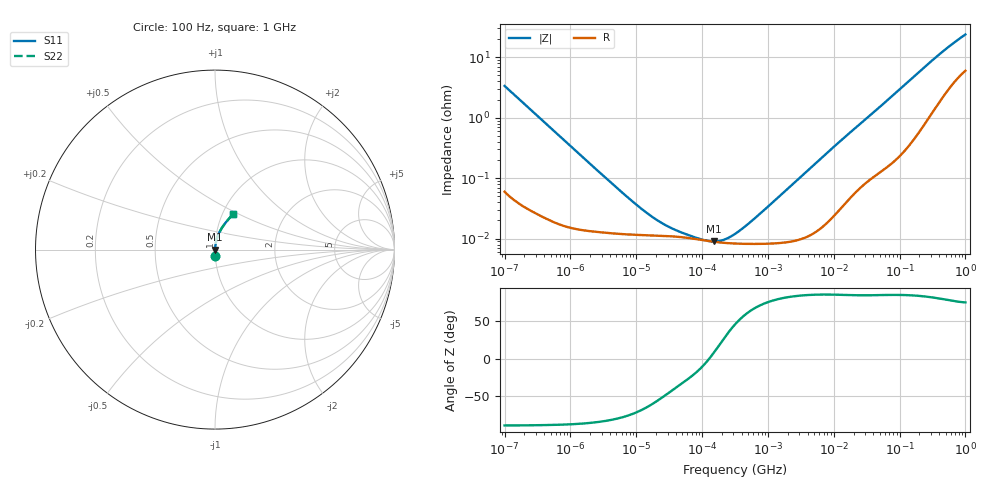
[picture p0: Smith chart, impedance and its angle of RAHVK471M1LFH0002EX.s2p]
! RAHVK471M1LFH0002EX  S-PARAMETER MODEL  (AEC-Q200 qualified)
! Model Generated by ELNA Corporation (http://www.ty-top.com)
! Version 1.0
! ELNA Control No. 201210
! Copyright (c) 2020 ELNA CO.,LTD. All Rights Reserved.
! Products Name : CONDUCTIVE POLYMER HYBRID ALUMINUM ELECTROLYTIC CAPACITORS
! Characteristics :
!  Capacitance  :  470uF  ,  Rated voltage  :  10V
!  Operating Temp. Range  :  -55 to +125 degC  ,  Endurance  :  4000hr at 125 degC
!  Dimension D  :  10mm  ,  Dimension L  :  10mm
! Frequency Range : 100Hz - 1GHz
! External Node Assignments :
!  1  o---| |---o  2
# MHz S RI R 50
!Freq[MHz].  S11 Real  S11 Imag  S21 Real  S21 Imag  S12 Real  S12 Imag  S22 Real  S22 Imag
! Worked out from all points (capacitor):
!   401 points, 100 Hz to 1 GHz, reference 50 ohm
!   read as one part in series: C = 473 uF near 108 Hz
!   lowest |Z| = 8.98 mohm at 153.1 kHz (marker M1)
!   series resonance near 127.7 kHz, so ESL is about 3.3 nH
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0.0001  0.00172 -0.0335  0.9983 0.0335  0.9983 0.0335  0.00172 -0.0335
0.000113  0.00141 -0.0297  0.9986 0.0297  0.9986 0.0297  0.00141 -0.0297
0.000309  0.000376 -0.0109  0.9996 0.0109  0.9996 0.0109  0.000376 -0.0109
0.001488  0.000144 -0.0023  0.9999 0.0023  0.9999 0.0023  0.000144 -0.0023
0.00876  0.000117 -0.000396  0.9999 0.000396  0.9999 0.000396  0.000117 -0.000396
0.014791  0.000114 -0.000235  0.9999 0.000235  0.9999 0.000235  0.000114 -0.000235
0.022131  0.000112 -0.000158  0.9999 0.000158  0.9999 0.000158  0.000112 -0.000158
0.038905  0.000108 -8.88e-05  0.9999 8.88e-05  0.9999 8.88e-05  0.000108 -8.88e-05
0.080353  9.85e-05 -3.3e-05  0.9999 3.3e-05  0.9999 3.3e-05  9.85e-05 -3.3e-05
0.094406  9.58e-05 -2.18e-05  0.9999 2.18e-05  0.9999 2.18e-05  9.58e-05 -2.18e-05
0.153109  8.87e-05 1.42e-05  0.9999 -1.42e-05  0.9999 -1.42e-05  8.87e-05 1.42e-05
0.238506  8.45e-05 5.44e-05  0.9999 -5.44e-05  0.9999 -5.44e-05  8.45e-05 5.44e-05
0.316228  8.3e-05 8.62e-05  0.9999 -8.62e-05  0.9999 -8.62e-05  8.3e-05 8.62e-05
0.436516  8.21e-05 0.000132  0.9999 -0.000132  0.9999 -0.000132  8.21e-05 0.000132
0.679986  8.19e-05 0.000218  0.9999 -0.000218  0.9999 -0.000218  8.19e-05 0.000218
4.704354  0.000121 0.00156  0.9999 -0.00156  0.9999 -0.00156  0.000121 0.00156
13.4122  0.000354 0.00436  0.9996 -0.00436  0.9996 -0.00436  0.000354 0.00436
69.9842  0.00205 0.0207  0.9979 -0.0207  0.9979 -0.0207  0.00205 0.0207
176.8072  0.0074 0.0505  0.9926 -0.0505  0.9926 -0.0505  0.0074 0.0505
380.1894  0.0266 0.1006  0.9734 -0.1006  0.9734 -0.1006  0.0266 0.1006
668.3439  0.0617 0.1533  0.9383 -0.1533  0.9383 -0.1533  0.0617 0.1533
1000  0.0992 0.1962  0.9008 -0.1962  0.9008 -0.1962  0.0992 0.1962
